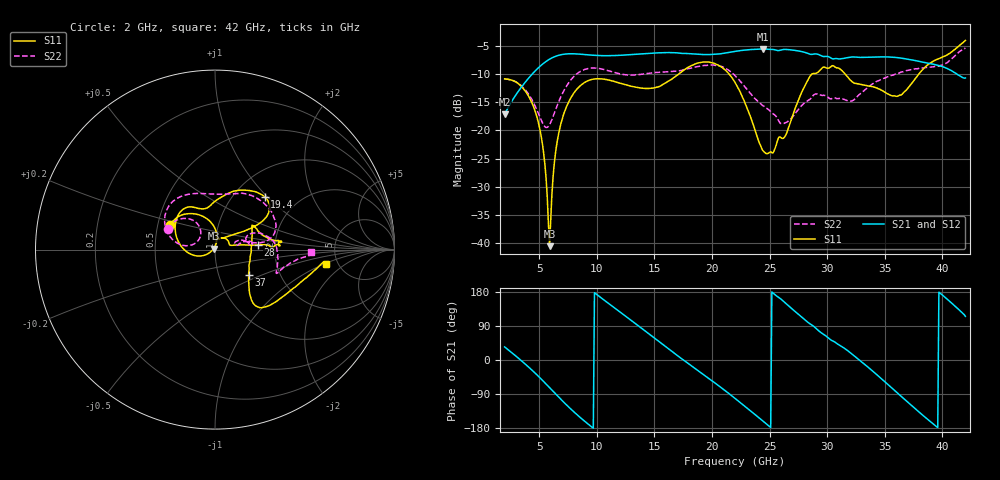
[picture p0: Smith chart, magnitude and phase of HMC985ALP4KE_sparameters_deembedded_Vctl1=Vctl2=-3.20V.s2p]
!s2p File: Measurements: S11, S21, S12, S22
# GHz S dB R 50.0
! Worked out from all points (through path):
!   401 points, 2 GHz to 42 GHz, reference 50 ohm
!   highest |S21| = -5.61 dB at 24.4 GHz (marker M1); lowest = -17.2 dB at 2 GHz (marker M2)
!   lowest |S11| = -40.5 dB at 5.9 GHz (marker M3), VSWR 1.02, Z = 49.2 + j0.521 ohm
!   |S11| at or under -10 dB: start of sweep to 17.13 GHz; 21.47 GHz to 28.69 GHz (7.221 GHz wide, 28.8 % of centre); 31.55 GHz to 37.97 GHz (6.419 GHz wide, 18.5 % of centre)
!   |S22| runs from -19.5 to -5.4 dB; largest |S21 - S12| = 0.00059
!   S11 on the Smith chart (normalised r, x): 2 GHz: 0.58, +0.17; 19.4 GHz: 1.37, +0.96; 28 GHz: 1.62, +0.09; 37 GHz: 1.39, -0.42; 42 GHz: 4.02, -1.08
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2  -10.88 151.2  -17.18 34.6  -17.18 34.6  -10.90 156.1
4.7  -16.92 95.9  -9.38 -36.1  -9.38 -36.1  -15.92 124.1
5.3  -22.63 81.5  -8.26 -54.1  -8.26 -54.1  -18.73 133.7
5.9  -40.50 145.9  -7.40 -72.8  -7.40 -72.8  -18.99 159.6
6.4  -24.28 -150.9  -6.91 -88.6  -6.91 -88.6  -16.49 171.5
6.9  -18.71 -163.1  -6.61 -104.2  -6.60 -104.2  -13.97 171.4
8.7  -11.87 150.6  -6.54 -155.2  -6.54 -155.2  -9.43 145.5
10.5  -10.90 125.6  -6.78 161.2  -6.78 161.2  -9.16 119.8
12.5  -11.92 113.9  -6.65 115.6  -6.65 115.6  -10.16 93.9
15.4  -12.25 96.9  -6.28 48.8  -6.28 48.8  -9.72 72.2
17.3  -9.75 75.9  -6.36 4.8  -6.36 4.8  -9.41 67.6
19.4  -7.89 46.8  -6.58 -41.6  -6.58 -41.6  -8.51 44.2
22  -11.50 30.4  -6.02 -101.3  -6.02 -101.3  -10.30 10.4
24.4  -23.53 65.8  -5.61 -160.4  -5.61 -160.4  -15.59 15.5
26.3  -21.18 16.7  -5.67 152.4  -5.67 152.4  -18.71 18.5
28  -12.38 6.3  -6.16 107.6  -6.16 107.6  -15.18 16.5
28.7  -9.98 1.5  -6.54 91.8  -6.55 91.8  -14.03 13.7
32.4  -11.67 23.5  -7.01 9.5  -7.01 9.4  -14.45 22.2
35.4  -13.66 9.2  -7.01 -68.0  -7.01 -68.1  -10.44 13.9
37  -12.56 -37.4  -7.40 -111.4  -7.40 -111.4  -9.38 3.7
39.4  -7.56 -50.2  -8.38 -173.4  -8.38 -173.5  -8.66 -21.0
42  -4.08 -7.5  -10.73 115.2  -10.73 115.2  -5.41 -1.4
